FUNCTION_BLOCK FB_LN_IED_LD1_LEDGGIO5 EXTENDS FB_AcsiCommonLogicalNodeClass
VAR_INPUT
	NamPlt: FB_DO_IED_LD1_LEDGGIO5_NamPlt := (sClass:='LPL', bLinkResult:=THIS^.AddDataToContainer(ipData:=NamPlt));
	Beh: FB_DO_IED_LD1_LEDGGIO5_Beh := (sClass:='ENS', bLinkResult:=THIS^.AddDataToContainer(ipData:=Beh));
	Health: FB_DO_IED_LD1_LEDGGIO5_Health := (sClass:='ENS', bLinkResult:=THIS^.AddDataToContainer(ipData:=Health));
	Mod_: FB_DO_IED_LD1_LEDGGIO5_Mod := (sObjectName:='Mod', sClass:='ENC', bLinkResult:=THIS^.AddDataToContainer(ipData:=Mod_));
	SPCSO1: FB_DO_IED_LD1_LEDGGIO5_SPCSO1 := (sClass:='SPC', bLinkResult:=THIS^.AddDataToContainer(ipData:=SPCSO1));
END_VAR
VAR
END_VAR

END_FUNCTION_BLOCK
